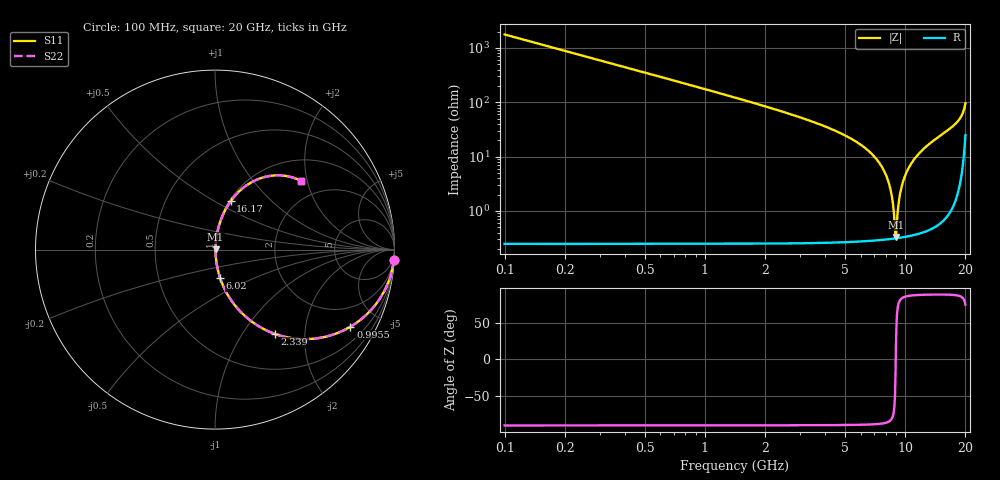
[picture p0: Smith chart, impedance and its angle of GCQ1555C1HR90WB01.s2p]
!Murata Part Number: GCQ1555C1HR90WB01
!These Parameters are Measured in Series Mode Connection
!Data Generated on Mar 13, 2026
!  o--ll--o
!Port1  Port2
!  o------o
!Operation Temp=25[degC], DC Bias Voltage=0[V]
!Freq. Start=100[MHz] Stop=20[GHz] 401[Steps]
# Hz S RI R 50
!Freq.(Hz) S11(Real) S11(Imag) S21(Real) S21(Imag) S12(Real) S12(Imag) S22(Real) S22(Imag)
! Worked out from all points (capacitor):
!   401 points, 100 MHz to 20 GHz, reference 50 ohm
!   read as one part in series: C = 900 fF near 199.5 MHz
!   lowest |Z| = 333 mohm at 9.005 GHz (marker M1)
!   series resonance near 8.981 GHz, so ESL is about 350 pH
!   S11 on the Smith chart (normalised r, x): 100 MHz: 1, -35; 995.5 MHz: 1.00, -3.51; 2.339 GHz: 1.01, -1.41; 6.02 GHz: 1.01, -0.33; 16.17 GHz: 1.02, +0.59; 20 GHz: 1.50, +1.84
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1e8  0.9968 -0.0564  0.0032 0.0564  0.0032 0.0564  0.9968 -0.0564
2.99e8  0.9721 -0.1645  0.0279 0.1645  0.0279 0.1645  0.9721 -0.1645
4.4825e8  0.9392 -0.2386  0.0608 0.2386  0.0608 0.2386  0.9392 -0.2386
9.955e8  0.7546 -0.4296  0.2454 0.4296  0.2454 0.4296  0.7546 -0.4296
2.33875e9  0.3334 -0.4696  0.6666 0.4696  0.6666 0.4696  0.3334 -0.4696
3.43325e9  0.1647 -0.368  0.8353 0.368  0.8353 0.368  0.1647 -0.368
6.02025e9  0.0287 -0.1589  0.9713 0.1589  0.9713 0.1589  0.0287 -0.1589
6.7665e9  0.0158 -0.1129  0.9842 0.1129  0.9842 0.1129  0.0158 -0.1129
7.662e9  0.00701 -0.0637  0.993 0.0637  0.993 0.0637  0.00701 -0.0637
8.259e9  0.00415 -0.0337  0.9958 0.0337  0.9958 0.0337  0.00415 -0.0337
8.60725e9  0.00336 -0.0172  0.9966 0.0172  0.9966 0.0172  0.00336 -0.0172
8.90575e9  0.00312 -0.00339  0.9969 0.00339  0.9969 0.00339  0.00312 -0.00339
9.00525e9  0.00313 0.00111  0.9969 -0.00111  0.9969 -0.00111  0.00313 0.00111
9.254e9  0.00332 0.0122  0.9967 -0.0122  0.9967 -0.0122  0.00332 0.0122
9.40325e9  0.00355 0.0187  0.9964 -0.0187  0.9964 -0.0187  0.00355 0.0187
1.005e10  0.00547 0.0461  0.9945 -0.0461  0.9945 -0.0461  0.00547 0.0461
1.13435e10  0.0132 0.0971  0.9868 -0.0971  0.9868 -0.0971  0.0132 0.0971
1.338325e10  0.0349 0.1711  0.9651 -0.1711  0.9651 -0.1711  0.0349 0.1711
1.616925e10  0.0873 0.2694  0.9127 -0.2694  0.9127 -0.2694  0.0873 0.2694
1.67165e10  0.103 0.2901  0.897 -0.2901  0.897 -0.2901  0.103 0.2901
1.885575e10  0.2245 0.3859  0.7755 -0.3859  0.7755 -0.3859  0.2245 0.3859
2e10  0.4813 0.3823  0.5187 -0.3823  0.5187 -0.3823  0.4813 0.3823
